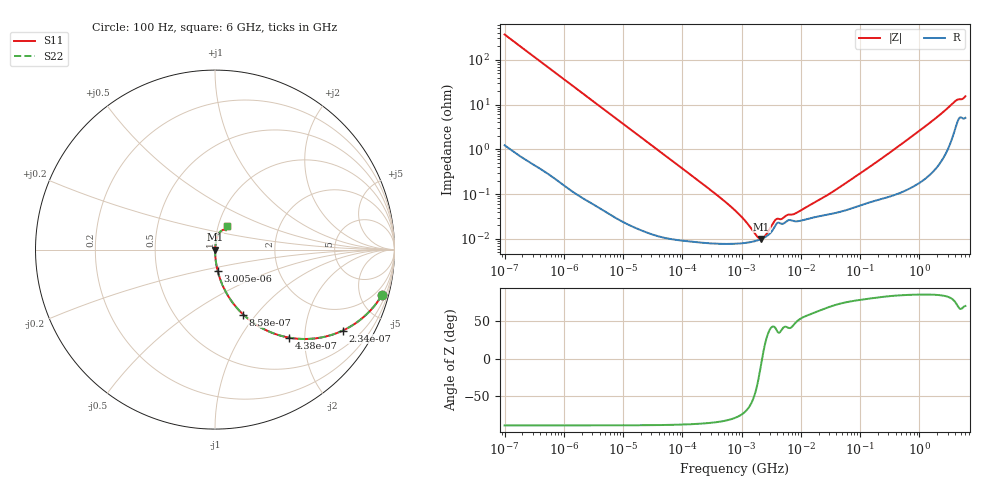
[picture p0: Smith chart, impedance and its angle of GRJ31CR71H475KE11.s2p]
!Murata Part Number: GRJ31CR71H475KE11
!These Parameters are Measured in Series Mode Connection
!Data Generated on Jun 19, 2026
!  o--ll--o
!Port1  Port2
!  o------o
!Operation Temp=25[degC], DC Bias Voltage=0[V]
!Freq. Start=100[Hz] Stop=6[GHz] 401[Steps]
# Hz S RI R 50
!Freq.(Hz) S11(Real) S11(Imag) S21(Real) S21(Imag) S12(Real) S12(Imag) S22(Real) S22(Imag)
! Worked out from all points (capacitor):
!   401 points, 100 Hz to 6 GHz, reference 50 ohm
!   read as one part in series: C = 4.33 uF near 109 Hz
!   lowest |Z| = 10 mohm at 2.169 MHz (marker M1)
!   series resonance near 2.224 MHz, so ESL is about 1.2 nH
!   S11 on the Smith chart (normalised r, x): 100 Hz: 1.02, -7.35; 234 Hz: 1.01, -3.14; 438 Hz: 1.01, -1.68; 858 Hz: 1.00, -0.86; 3.005 kHz: 1.00, -0.25; 6 GHz: 1.10, +0.29
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100  0.9303 -0.253  0.0697 0.253  0.0697 0.253  0.9303 -0.253
150  0.8571 -0.3483  0.1429 0.3483  0.1429 0.3483  0.8571 -0.3483
234  0.7112 -0.4514  0.2888 0.4514  0.2888 0.4514  0.7112 -0.4514
438  0.4146 -0.4906  0.5854 0.4906  0.5854 0.4906  0.4146 -0.4906
858  0.1574 -0.3621  0.8426 0.3621  0.8426 0.3621  0.1574 -0.3621
2008  0.0336 -0.1779  0.9664 0.1779  0.9664 0.1779  0.0336 -0.1779
3005  0.0155 -0.1213  0.9845 0.1213  0.9845 0.1213  0.0155 -0.1213
8416  0.00221 -0.044  0.9978 0.044  0.9978 0.044  0.00221 -0.044
40335  0.000199 -0.00925  0.9998 0.00925  0.9998 0.00925  0.000199 -0.00925
774597  7.81e-05 -0.000427  0.9999 0.000427  0.9999 0.000427  7.81e-05 -0.000427
1159002  8.13e-05 -0.000237  0.9999 0.000237  0.9999 0.000237  8.13e-05 -0.000237
1813585  9.16e-05 -7e-05  0.9999 7e-05  0.9999 7e-05  9.16e-05 -7e-05
2169299  9.97e-05 -8.5e-06  0.9999 8.5e-06  0.9999 8.5e-06  9.97e-05 -8.5e-06
2481164  0.000109 3.8e-05  0.9999 -3.8e-05  0.9999 -3.8e-05  0.000109 3.8e-05
3882480  0.000217 0.000174  0.9998 -0.000174  0.9998 -0.000174  0.000217 0.000174
7947587  0.000247 0.000268  0.9998 -0.000268  0.9998 -0.000268  0.000247 0.000268
1.555665e7  0.000296 0.000527  0.9997 -0.000527  0.9997 -0.000527  0.000296 0.000527
4.35672e7  0.000396 0.00132  0.9996 -0.00132  0.9996 -0.00132  0.000396 0.00132
3.124326e8  0.000943 0.00826  0.9991 -0.00826  0.9991 -0.00826  0.000943 0.00826
1.497423e9  0.00415 0.0385  0.9958 -0.0385  0.9958 -0.0385  0.00415 0.0385
4.009986e9  0.0391 0.1072  0.9609 -0.1072  0.9609 -0.1072  0.0391 0.1072
6e9  0.0658 0.1288  0.9342 -0.1288  0.9342 -0.1288  0.0658 0.1288
